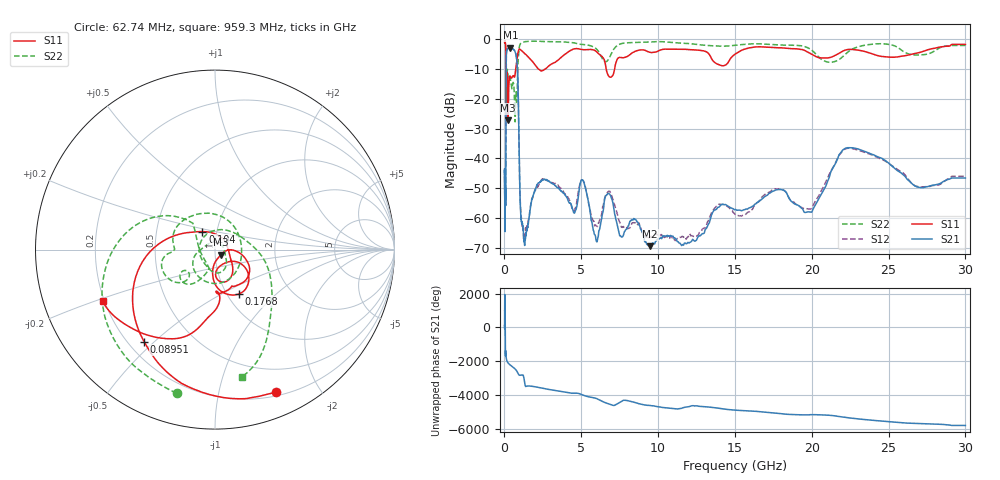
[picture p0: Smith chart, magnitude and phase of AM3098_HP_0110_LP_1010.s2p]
! Date/Time: Thu, Feb 28, 2019 8:37 AM
! Network Analyzer: Agilent Technologies E8364B Rev: A.07.50.67
! Sweep from 0.010 to 30.000 GHz, 1601 Points, Sweep Type: LOG
! Power Supply: 5.022 V, 0.002 A
# Hz S DB R 50
!freq MagS11 AngS11 MagS21 AngS21 MagS12 AngS12 MagS22 AngS22
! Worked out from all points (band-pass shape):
!   1601 points, 10 MHz to 30 GHz, reference 50 ohm
!   highest |S21| = -2.82 dB at 382 MHz (marker M1); lowest = -69.5 dB at 9.49 GHz (marker M2)
!   |S21| within 3 dB of the highest: 118.1 MHz to 772.9 MHz (654.8 MHz wide, 147 % of centre)
!   lowest |S11| = -27.2 dB at 238.7 MHz (marker M3), VSWR 1.09, Z = 53.3 - j3.1 ohm
!   |S11| at or under -10 dB: 99.92 MHz to 731.1 MHz (631.2 MHz wide, 152 % of centre); 2.222 GHz to 2.646 GHz (424.1 MHz wide, 17.4 % of centre); 6.624 GHz to 7.169 GHz (544.8 MHz wide, 7.9 % of centre)
!   |S22| runs from -27.7 to -0.6 dB; largest |S21 - S12| = 0.013
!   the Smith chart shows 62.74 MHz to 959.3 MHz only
!   S11 on the Smith chart (normalised r, x): 62.74 MHz: 0.24, -1.49; 89.51 MHz: 0.26, -0.46; 104 MHz: 0.85, +0.17; 176.8 MHz: 1.14, -0.61; 959.3 MHz: 0.19, -0.21
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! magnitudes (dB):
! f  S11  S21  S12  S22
! 10 MHz  -0.3  -44.0  -44.9  -0.6
! 38.04 MHz  -0.5  -63.6  -58.7  -0.9
! 62.74 MHz  -1.3  -53.8  -53.8  -1.7
! 89.51 MHz  -3.8  -41.3  -41.1  -4.1
! 104 MHz  -18.2  -12.6  -12.6  -21.1
! 144.7 MHz  -18.9  -3.8  -3.8  -14.1
! 176.8 MHz  -11.0  -3.5  -3.4  -10.1
! 238.7 MHz  -27.2  -2.9  -2.9  -12.5
! 382 MHz  -12.5  -2.8  -2.8  -13.2
! 550.5 MHz  -12.3  -3.3  -3.2  -14.6
! 825.6 MHz  -6.3  -8.5  -8.5  -17.9
! 959.3 MHz  -3.2  -38.5  -38.7  -2.8
! 1.302 GHz  -4.7  -68.4  -66.6  -0.8
! 2.084 GHz  -9.2  -49.3  -50.2  -0.6
! 5.103 GHz  -3.4  -47.3  -47.5  -1.7
! 5.929 GHz  -3.9  -66.3  -62.4  -2.9
! 6.753 GHz  -12.1  -51.8  -51.2  -6.8
! 7.926 GHz  -5.9  -63.8  -63.5  -1.2
! 9.49 GHz  -4.4  -69.5  -66.6  -0.9
! 19.7 GHz  -4.2  -58.0  -56.9  -2.7
! 22.67 GHz  -3.4  -36.5  -36.7  -3.2
! 30 GHz  -1.7  -46.6  -46.0  -2.0
